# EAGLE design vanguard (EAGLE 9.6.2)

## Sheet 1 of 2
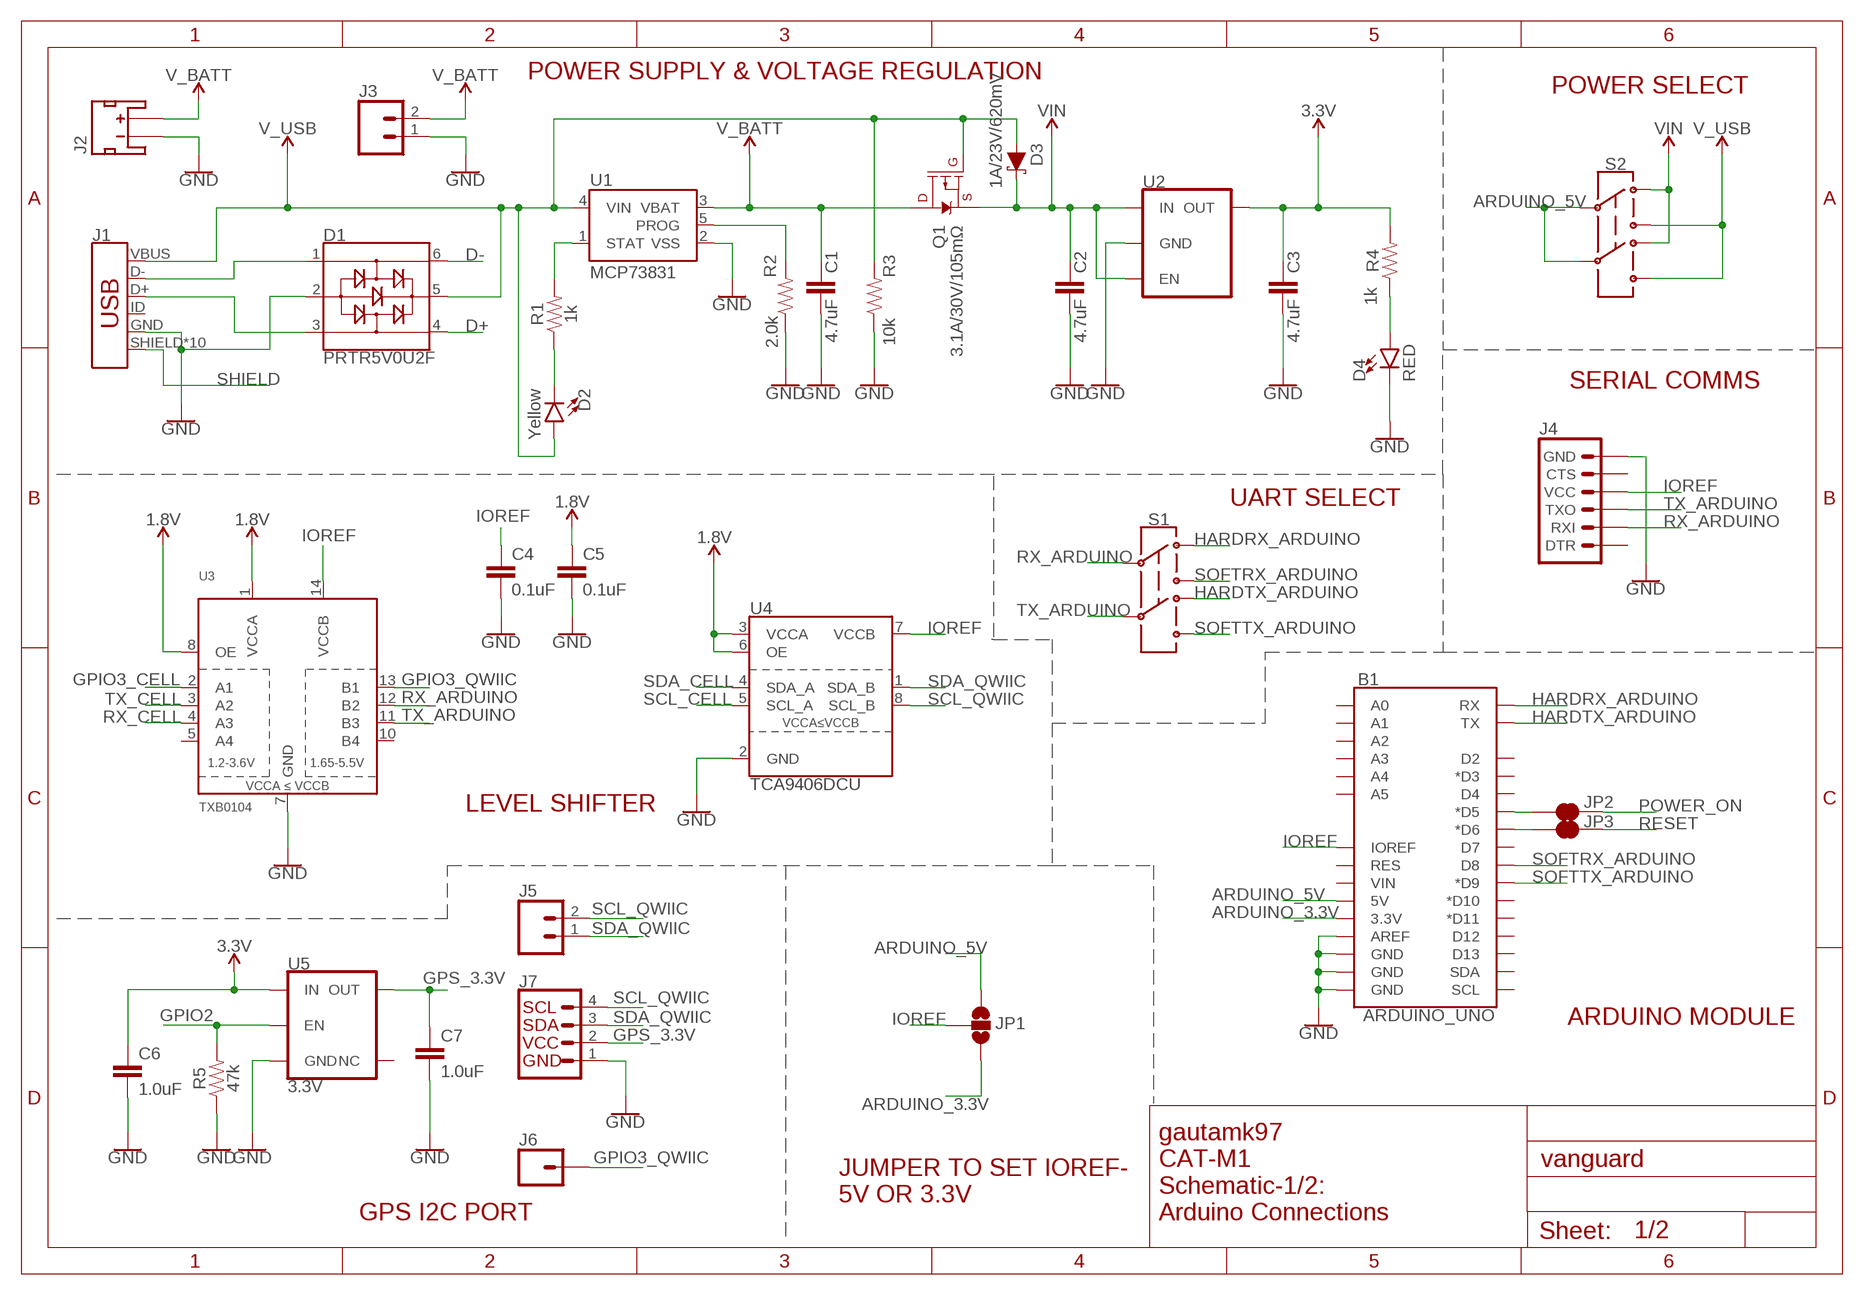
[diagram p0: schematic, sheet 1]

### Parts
B1  ARDUINO_UNO  ARDUINO_UNO_R3_SHIELDNOLABELS  [UNO_R3_SHIELD_NOLABELS]
C1  4.7uF  4.7UF-0603-6.3V-(10%)  [0603]
C2  4.7uF  4.7UF-0603-6.3V-(10%)  [0603]
C3  4.7uF  4.7UF-0603-6.3V-(10%)  [0603]
C4  0.1uF  0.1UF-0603-25V-(+80/-20%)  [0603]
C5  0.1uF  0.1UF-0603-25V-(+80/-20%)  [0603]
C6  1.0uF  1.0UF-0603-16V-10%  [0603]
C7  1.0uF  1.0UF-0603-16V-10%  [0603]
D1  PRTR5V0U2F  [SOT886]
D2  Yellow  LED-YELLOW0603  [LED-0603]
D3  1A/23V/620mV  DIODE-SCHOTTKY-BAT20J  [SOD-323]
D4  RED  LED-RED0603  [LED-0603]
J1  USB_MICRO-B_HALF_PTH_MILL  [USB-MICROB-PTH-MILL]
J2  JST_2MM_MALE  [JST-2-SMD]
J3  CONN_021X02_NO_SILK  [1X02_NO_SILK]
J4  6_PIN_SERIAL_TARGET_NO_SILK  [1X06_NO_SILK]
J5  CONN_021X02_NO_SILK  [1X02_NO_SILK]
J6  CONN_01PTH_NO_SILK_YES_STOP  [1X01_NO_SILK]
J7  QWIIC_CONNECTORJS-1MM  [JST04_1MM_RA]
JP1  JUMPER-SMT_3_NO_SILK  [SMT-JUMPER_3_NO_SILK]
JP2  JUMPER-SMT_2_NC_TRACE_SILK  [SMT-JUMPER_2_NC_TRACE_SILK]
JP3  JUMPER-SMT_2_NC_TRACE_SILK  [SMT-JUMPER_2_NC_TRACE_SILK]
Q1  3.1A/30V/105mΩ  MOSFET_PCH-DMG2307L  [SOT23-3]
R1  1k  1KOHM-0603-1/10W-1%  [0603]
R2  2.0k  2.0KOHM-0603-1/10W-5%  [0603]
R3  10k  10KOHM-0603-1/10W-1%  [0603]
R4  1k  1KOHM-0603-1/10W-1%  [0603]
R5  47k  47KOHM-0603-1/10W-1%  [0603]
S1  SWITCH-DPDT-SMD-AYZ0202  [SWITCH_DPDT_SMD_AYZ0202]
S2  SWITCH-DPDT-SMD-AYZ0202  [SWITCH_DPDT_SMD_AYZ0202]
U1  MCP73831  [SOT23-5]
U2  AP7361C-33FGEUDFN-8  [UDFN-8]
U3  TXB0104  TXB0104PWR  [TSSOP14]
U4  TCA9406DCU  [VSSOP-8]
U5  3.3V  V_REG_AP2112K-3.3V  [SOT23-5]

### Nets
1.8V: C5.1 U3.1(VCCA) U3.8(OE) U4.3(VCCA) U4.6(OE) ; also sheet 2
3.3V: C3.1 C6.1 R4.2 U2.1(OUT) U5.1(IN) ; also sheet 2
ARDUINO_3.3V: B1.3.3V JP1.3
ARDUINO_5V: B1.5V JP1.1 S2.2 S2.5
D+: D1.4 ; also sheet 2
D-: D1.6 ; also sheet 2
GND: B1.AREF B1.GND@0(GND) B1.GND@1(GND) B1.GND@2(GND) C1.2 C2.2 C3.2 C4.2 C5.2 C6.2 C7.2 D1.2 D4.C J1.GND J2.1(-) J3.1 J4.6(GND) J7.1 R2.1 R3.1 R5.1 U1.2(VSS) U2.4(GND) U2.EP(GND) U3.7(GND) U4.2(GND) U5.2(GND) ; also sheet 2
GPIO2: R5.2 U5.3(EN) ; also sheet 2
GPIO3_CELL: U3.2(A1)
GPIO3_QWIIC: J6.1 U3.13(B1)
GPS_3.3V: C7.1 J7.2 U5.5(OUT)
HARDRX_ARDUINO: B1.RX S1.3
HARDTX_ARDUINO: B1.TX S1.6
IOREF: B1.IOREF C4.1 J4.4(VCC) JP1.2 U3.14(VCCB) U4.7(VCCB)
N$1: D1.1 J1.D-
N$3: D1.3 J1.D+
N$4: D4.A R4.1
N$6: R1.2 U1.1(STAT)
N$7: D2.C R1.1
N$9: B1.D5(*D5) JP2.1
N$10: R2.2 U1.5(PROG)
N$11: B1.D6(*D6) JP3.1
POWER_ON: JP2.2
RESET: JP3.2
RX_ARDUINO: J4.2(RXI) S1.2 U3.12(B2)
RX_CELL: U3.4(A3) ; also sheet 2
SCL_CELL: U4.5(SCL_A) ; also sheet 2
SCL_QWIIC: J5.2 J7.4 U4.8(SCL_B)
SDA_CELL: U4.4(SDA_A) ; also sheet 2
SDA_QWIIC: J5.1 J7.3 U4.1(SDA_B)
SHIELD: J1.SHIELD J1.SHIELD2(SHIELD) J1.SHIELD3(SHIELD) J1.SHIELD4(SHIELD) J1.SHIELD5(SHIELD) J1.SHIELD6(SHIELD) J1.SHIELD7(SHIELD) J1.SHIELD8(SHIELD) J1.SHIELD9(SHIELD) J1.SHIELD10(SHIELD)
SOFTRX_ARDUINO: B1.D8 S1.1
SOFTTX_ARDUINO: B1.D9(*D9) S1.4
TX_ARDUINO: J4.3(TXO) S1.5 U3.11(B3)
TX_CELL: U3.3(A2) ; also sheet 2
V_BATT: C1.1 J2.2(+) J3.2 Q1.3(D) U1.3(VBAT)
V_USB: D1.5 D2.A D3.A J1.VBUS Q1.1(G) R3.2 S2.1 S2.4 U1.4(VIN) ; also sheet 2
VIN: C2.1 D3.C Q1.2(S) S2.3 S2.6 U2.5(EN) U2.8(IN)
Unconnected: B1.A0 B1.A1 B1.A2 B1.A3 B1.A4 B1.A5 B1.D2 B1.D3(*D3) B1.D4 B1.D7 B1.D10(*D10) B1.D11(*D11) B1.D12 B1.D13 B1.RES B1.SCL B1.SDA B1.VIN J1.ID J2.NC1(PAD1) J2.NC2(PAD2) J4.1(DTR) J4.5(CTS) U3.5(A4) U3.10(B4) U5.4(NC)

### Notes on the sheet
- POWER SUPPLY & VOLTAGE REGULATION
- POWER SELECT
- SERIAL COMMS
- UART SELECT
- LEVEL SHIFTER
- ARDUINO MODULE
- JUMPER TO SET IOREF- 
  5V OR 3.3V
- GPS I2C PORT
- gautamk97
  CAT-M1
  Schematic-1/2: 
  Arduino Connections

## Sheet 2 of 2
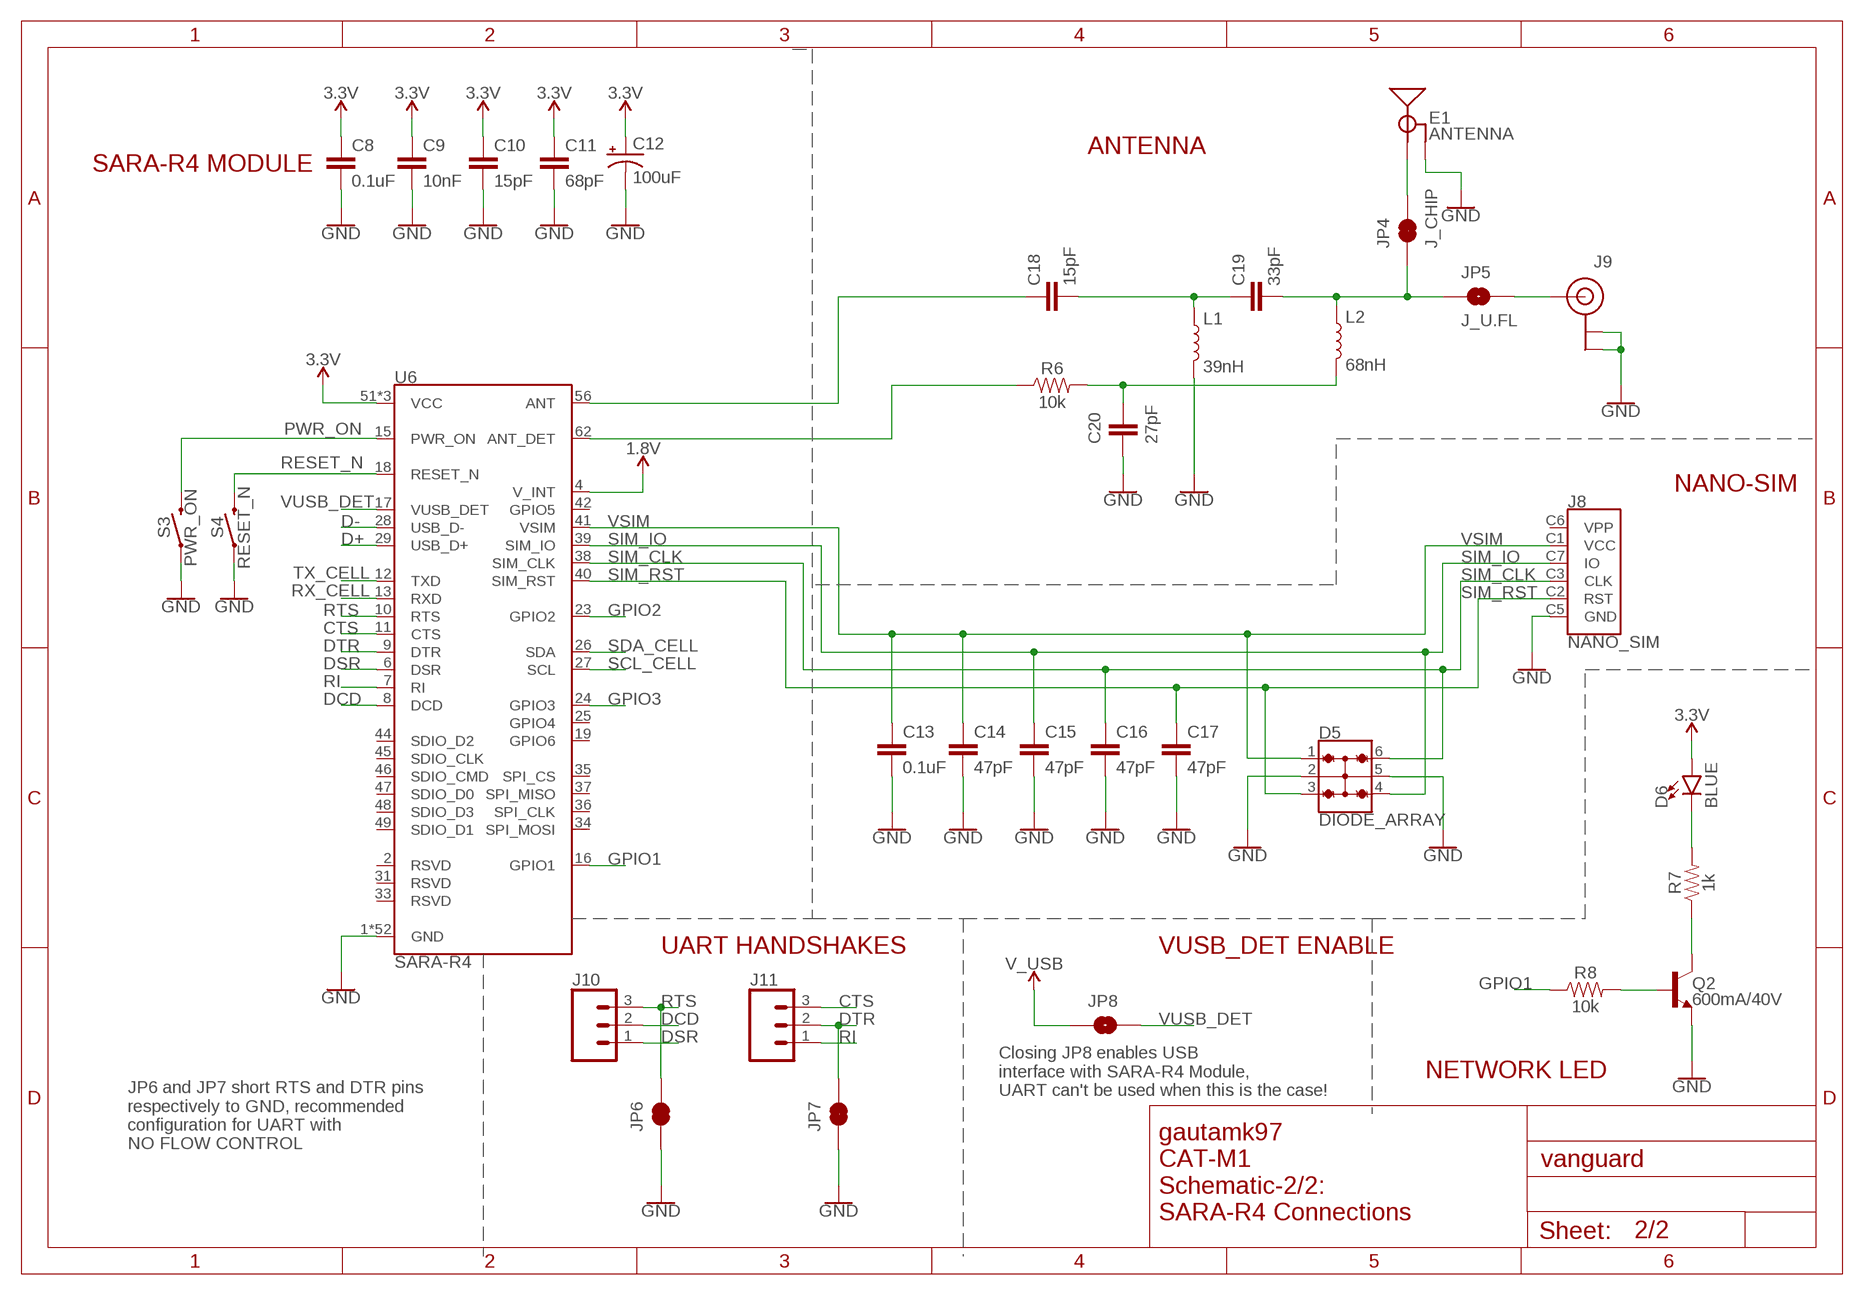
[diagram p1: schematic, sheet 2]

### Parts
C8  0.1uF  0.1UF-0603-25V-(+80/-20%)  [0603]
C9  10nF  10NF-0603-50V-10%  [0603]
C10  15pF  15PF-0603-50V-5%  [0603]
C11  68pF  68PF-0603-50V-5%  [0603]
C12  100uF  100UF-POLAR-1206-6.3V-20%  [1206-POLAR]
C13  0.1uF  0.1UF-0603-25V-(+80/-20%)  [0603]
C14  47pF  47PF-0603-50V-5%  [0603]
C15  47pF  47PF-0603-50V-5%  [0603]
C16  47pF  47PF-0603-50V-5%  [0603]
C17  47pF  47PF-0603-50V-5%  [0603]
C18  15pF  15PF-0603-50V-5%  [0603]
C19  33pF  33PF-0603-50V-5%  [0603]
C20  27pF  27PF-0603-50V-5%  [0603]
D5  DIODE_ARRAY  TVS_DIODE_ARRAY_4DT1042-04SO-7  [SOT23-6L]
D6  BLUE  LED-BLUE0603  [LED-0603]
E1  ANTENNA  ANTENNA-GROUNDEDMOLEX-146200  [MOLEX_146200]
J8  NANO_SIM  NANO_SIMWURTH  [NANO_SIM_WURTH_693043020611]
J9  U.FL  [U.FL]
J10  CONN_031X03_NO_SILK  [1X03_NO_SILK]
J11  CONN_031X03_NO_SILK  [1X03_NO_SILK]
JP4  J_CHIP  JUMPER-SMT_2_NC_TRACE_NO-SILK  [SMT-JUMPER_2_NC_TRACE_NO-SILK]
JP5  J_U.FL  JUMPER-SMT_2_NO_NO-SILK  [SMT-JUMPER_2_NO_NO-SILK]
JP6  JUMPER-SMT_2_NC_TRACE_SILK  [SMT-JUMPER_2_NC_TRACE_SILK]
JP7  JUMPER-SMT_2_NC_TRACE_SILK  [SMT-JUMPER_2_NC_TRACE_SILK]
JP8  JUMPER-SMT_2_NO_SILK  [SMT-JUMPER_2_NO_SILK]
L1  39nH  INDUCTOR-0603-39NH  [0603]
L2  68nH  INDUCTOR-0603-68NH  [0603]
Q2  600mA/40V  TRANS_NPN-MMBT2222AL  [SOT23-3]
R6  10k  10KOHM-0603-1/10W-1%  [0603]
R7  1k  1KOHM-0603-1/10W-1%  [0603]
R8  10k  10KOHM-0603-1/10W-1%  [0603]
S3  PWR_ON  MOMENTARY-SWITCH-SPST-SMD-5.2MM-TALL  [TACTILE_SWITCH_SMD_5.2MM]
S4  RESET_N  MOMENTARY-SWITCH-SPST-SMD-5.2MM-TALL  [TACTILE_SWITCH_SMD_5.2MM]
U6  SARA-R4  [SARA-LGA]

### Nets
1.8V: U6.4(V_INT) ; also sheet 1
3.3V: C8.1 C9.1 C10.1 C11.1 C12.1(+) D6.A U6.51(VCC) U6.52(VCC) U6.53(VCC) ; also sheet 1
CTS: J11.3 U6.11(CTS)
D+: U6.29(USB_D+) ; also sheet 1
D-: U6.28(USB_D-) ; also sheet 1
DCD: J10.2 U6.8(DCD)
DSR: J10.1 U6.6(DSR)
DTR: J11.2 JP7.2 U6.9(DTR)
GND: C8.2 C9.2 C10.2 C11.2 C12.2(-) C13.2 C14.2 C15.2 C16.2 C17.2 C20.2 D5.2 D5.5 E1.GND J8.C5(GND) J9.1(GND) J9.2(GND) JP6.1 JP7.1 L1.2 Q2.2(E) S3.1 S4.1 U6.1(GND) U6.3(GND) U6.5(GND) U6.14(GND) U6.20(GND) U6.21(GND) U6.22(GND) U6.30(GND) U6.32(GND) U6.43(GND) U6.50(GND) U6.54(GND) U6.55(GND) U6.57(GND) U6.58(GND) U6.59(GND) U6.60(GND) U6.61(GND) U6.63(GND) U6.64(GND) U6.65(GND) U6.66(GND) U6.67(GND) U6.68(GND) U6.69(GND) U6.70(GND) U6.71(GND) U6.72(GND) U6.73(GND) U6.74(GND) U6.75(GND) U6.76(GND) U6.77(GND) U6.78(GND) U6.79(GND) U6.80(GND) U6.81(GND) U6.82(GND) U6.83(GND) U6.84(GND) U6.85(GND) U6.86(GND) U6.87(GND) U6.88(GND) U6.89(GND) U6.90(GND) U6.91(GND) U6.92(GND) U6.93(GND) U6.94(GND) U6.95(GND) U6.96(GND) ; also sheet 1
GPIO1: R8.1 U6.16(GPIO1)
GPIO2: U6.23(GPIO2) ; also sheet 1
GPIO3: U6.24(GPIO3)
N$8: R6.1 U6.62(ANT_DET)
N$12: C18.1 U6.56(ANT)
N$13: C18.2 C19.1 L1.1
N$14: C20.1 L2.2 R6.2
N$15: C19.2 JP4.1 JP5.1 L2.1
N$16: E1.FEED(SIGNAL) JP4.2
N$17: D6.C R7.2
N$18: J9.FEED(SIGNAL) JP5.2
N$19: Q2.1(B) R8.2
N$20: Q2.3(C) R7.1
PWR_ON: S3.3 U6.15(PWR_ON)
RESET_N: S4.3 U6.18(RESET_N)
RI: J11.1 U6.7(RI)
RTS: J10.3 JP6.2 U6.10(RTS)
RX_CELL: U6.13(RXD) ; also sheet 1
SCL_CELL: U6.27(SCL) ; also sheet 1
SDA_CELL: U6.26(SDA) ; also sheet 1
SIM_CLK: C16.1 D5.6 J8.C3(CLK) U6.38(SIM_CLK)
SIM_IO: C15.1 D5.4 J8.C7(IO) U6.39(SIM_IO)
SIM_RST: C17.1 D5.3 J8.C2(RST) U6.40(SIM_RST)
TX_CELL: U6.12(TXD) ; also sheet 1
V_USB: JP8.1 ; also sheet 1
VSIM: C13.1 C14.1 D5.1 J8.C1(VCC) U6.41(VSIM)
VUSB_DET: JP8.2 U6.17(VUSB_DET)
Unconnected: J8.C6(VPP) U6.2(RSVD) U6.19(GPIO6) U6.25(GPIO4) U6.31(RSVD) U6.33(RSVD) U6.34(SPI_MOSI) U6.35(SPI_CS) U6.36(SPI_CLK) U6.37(SPI_MISO) U6.42(GPIO5) U6.44(SDIO_D2) U6.45(SDIO_CLK) U6.46(SDIO_CMD) U6.47(SDIO_D0) U6.48(SDIO_D3) U6.49(SDIO_D1)

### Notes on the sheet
- ANTENNA
- SARA-R4 MODULE
- NANO-SIM
- UART HANDSHAKES | VUSB_DET ENABLE
- NETWORK LED
- Closing JP8 enables USB 
  interface with SARA-R4 Module, 
  UART can't be used when this is the case!
- JP6 and JP7 short RTS and DTR pins 
  respectively to GND, recommended 
  configuration for UART with 
  NO FLOW CONTROL
- gautamk97
  CAT-M1
  Schematic-2/2:
  SARA-R4 Connections

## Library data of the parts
B1 = SparkFun-Boards:ARDUINO_UNO_R3_SHIELD: Arduino R3 Shield Footprint Shield form compatible with the Arduino Uno R3. SparkFun Products: MG2639 Cellular Shield MIDI Shield R3 Stackable Headers Kit
C1-C3 = SparkFun-Capacitors:4.7UF: 4.7µF ceramic capacitors; PROD_ID: CAP-08280
C4 C5 C8 C13 = SparkFun-Capacitors:0.1UF: 0.1µF ceramic capacitors; PROD_ID: CAP-00810
C6 C7 = SparkFun-Capacitors:1.0UF: 1µF ceramic capacitors; PROD_ID: CAP-00868
C9 = SparkFun-Capacitors:10NF: 0.01uF/10nF/10,000pF ceramic capacitors; PROD_ID: CAP-00867
C10 C18 = SparkFun-Capacitors:15PF: 15pF ceramic capacitors; PROD_ID: CAP-07881
C11 = SparkFun-Capacitors:68PF: 68pF ceramic capacitors; PROD_ID: CAP-14092
C12 = ublox:100UF-POLAR: 100µF polarized capacitors; PROD_ID: CAP-14093
C14-C17 = SparkFun-Capacitors:47PF: 47pF ceramic capacitors; PROD_ID: CAP-08913
C19 = SparkFun-Capacitors:33PF: 33pF ceramic capacitors; PROD_ID: CAP-10142
C20 = SparkFun-Capacitors:27PF: 27pF ceramic capacitors; PROD_ID: CAP-09989
D1 = SparkFun-IC-Power:PRTR5V0U2: A small ESD protection device. Most commonly used on USB D+/D- signals to protect large, expensive, or especially sensitive USB enabled devices.; PROD_ID: DIO-14084
D2 = SparkFun-LED:LED-YELLOW: Yellow SMD LED; PROD_ID: DIO-09003
D3 = SparkFun-DiscreteSemi:DIODE-SCHOTTKY: Schottky diode; PROD_ID: DIO-11623
D4 = SparkFun-LED:LED-RED: Red SMD LED; PROD_ID: DIO-00819
D5 = ublox:TVS_DIODE_ARRAY_4; PROD_ID: DIO-14095
D6 = SparkFun-LED:LED-BLUE: Blue SMD LED; PROD_ID: DIO-08575
E1 = ublox:ANTENNA-GROUNDED: Antenna w/ Ground Connection; PROD_ID: ANT-14096
J1 = SparkFun-Connectors:USB_MICRO-B: USB Type Micro-B Connector Male/female and PTH/SMT variants SparkFun Products: SparkFun microB USB Breakout SparkFun USB microB Plug Breakout SparkFun ESP8266 Thing; PROD_ID: CONN-13711
J2 = SparkFun-Connectors:JST_2MM_MALE: JST 2MM MALE RA CONNECTOR Two pin, compact surface mount connector. Commonly used as a battery input connection point. We really like the solid locking feeling and high current rating on these small connectors. We use these all the time as battery connectors. Mates to single-cell LiPo batteries.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; PROD_ID: CONN-11443; SF_ID: PRT-08612
J3 J5 = SparkFun-Connectors:CONN_02: Multi connection point. Often used as Generic Header-pin footprint for 0.1 inch spaced/style header connections
J4 = SparkFun-Connectors:6_PIN_SERIAL_TARGET: 6-pin header connection for use with the "FTDI BASIC" pinout - TARGET SIDE. Also known as "Arduino Serial Program Header". It is used to mate with our FTDI Basic serial programmers using the Arduino IDE. Note, this device has "TARGET" in the name. It is intended to be used on a design that contains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
J6 = SparkFun-Connectors:CONN_01: Single connection point. Often used as Generic Header-pin footprint for 0.1 inch spaced/style header connections
J7 = SparkFun-Connectors:QWIIC_CONNECTOR: SparkFun I2C Standard Qwiic Connector An SMD 1mm pitch JST connector makes it easy and quick (get it? Qwiic?) to connect I2C devices to each other. The Qwiic system enables fast and solderless connection between popular platforms and various sensors and actuators. We carry 200mm, 100mm, 50mm, and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; PROD_ID: CONN-13694; VALUE: QWIIC_RIGHT_ANGLE
J8 = ublox:NANO_SIM; PROD_ID: CONN-14097
J9 = SparkFun-Connectors:U.FL: SMD Antenna Connector - U.FL 2mm height, 3.0mm x 3.0mm receptacle size. SparkFun Products: SparkFun WiFi Shield - ESP8266 SparkFun ESP8266 Thing SparkFun MiniGen - Pro Mini Signal Generator Shield; PROD_ID: CONN-09193; SF_ID: WRL-09144
J10 J11 = SparkFun-Connectors:CONN_03: Multi connection point. Often used as Generic Header-pin footprint for 0.1 inch spaced/style header connections On any of the 0.1 inch spaced packages, you can populate with these: Break Away Headers - Straight (PRT-00116) Break Away Male Headers - Right Angle (PRT-00553) Female Headers (PRT-00115)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
JP1 = SparkFun-Jumpers:JUMPER-SMT_3_NO: Normally open jumper This jumper has three pads in close proximity to each other. Apply solder to close the connection(s).
JP2-JP4 JP6 JP7 = SparkFun-Jumpers:JUMPER-SMT_2_NC_TRACE: Normally closed trace jumper
JP5 JP8 = SparkFun-Jumpers:JUMPER-SMT_2_NO: Normally open jumper
L1 = ublox:INDUCTOR: Inductors; PROD_ID: NDUC-14091
L2 = ublox:INDUCTOR: Inductors
Q1 = SparkFun-DiscreteSemi:MOSFET_PCH: P-channel MOSFETs Voltage controlled devices that allow control of high current outputs. SparkFun Products: SparkFun ESP32 Thing SparkFun ESP8266 Thing SparkFun Pi Servo HAT V2 DMG2305UX-7 (20V/4.2A/SOT23-3); PROD_ID: TRANS-11308
Q2 = SparkFun-DiscreteSemi:TRANS_NPN: NPN transistor Current controlled devices typically used to amplify current or used as a switch. BC547 - COM-08928 (TO-92 45V 100mA) (1.Collector 2.Base 3.Emitter) 2N3904 - COM-00521 (TO-92 40V 200mA) (1.Emitter 2.Base 3.Collector) P2N2222A - COM-12852 (TO-92 40V 600mA) (1.Collector 2.Base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; PROD_ID: TRANS-08049
R1 R4 R7 = SparkFun-Resistors:1KOHM: 1kΩ resistor; PROD_ID: RES-07856
R2 = SparkFun-Resistors:2.0KOHM: 2kΩ resistor; PROD_ID: RES-08296
R3 R6 R8 = SparkFun-Resistors:10KOHM: 10kΩ resistor; PROD_ID: RES-00824
R5 = SparkFun-Resistors:47KOHM: 47kΩ resistor; PROD_ID: RES-07871
S1 S2 = SparkFun-Switches:SWITCH-DPDT: Double-Pole, Double-Throw (DPDT) Switch Double-pole, double-throw switches. Variant Overview PTH-GPI-152-3013 Used on SparkFun Geiger Counter SMD-AY0202 Surface Mount DPDT Switch (COM-00597) Used on e.g. LilyPad Arduino USB - ATmega32U4 Board; PROD_ID: SWCH-08179; SF_SKU: COM-00597
S3 S4 = SparkFun-Switches:MOMENTARY-SWITCH-SPST: Momentary Switch (Pushbutton) - SPST; PROD_ID: SWCH-14139
U1 = SparkFun-IC-Power:MCP73831: MCP73831T Li-Ion, Li-Pol Controller Miniature single cell, fully integrated Li-Ion, Li-polymer charge management controller Datasheet SparkFun Products: SparkFun ESP32 Thing SparkFun 9DoF Razor IMU M0; PROD_ID: IC-09995
U2 = SparkFun-IC-Power:AP7361C-33FGE: AP7361C 3.3V LDO Regulator; PROD_ID: VREG-14094
U3 = SparkFun-IC-Comms:TXB0104PWR: 4-Bit Bi-Directional Level Shifter 1.2V-3.6V (VCCA) to 1.65V-5.5V (VCCB) bi-directional level shifter with auto direction sensing. Max data rate - VCCA 1.8V: 20Mbps (50ns), VCCA 3.3V: 100Mbps (10ns) Digikey: 296-21929-1-ND (TSSOP) Datasheet SparkFun Products SparkFun Cellular Shield - MG2639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; PROD_ID: IC-13929
U4 = ublox:TCA9406; PROD_ID: IC-14098
U5 = SparkFun-IC-Power:V_REG_AP2112: AP2112 - 600mA CMOS LDO Regulator w/ Enable The AP2112 is CMOS process low dropout linear regulator with enable function, the regulator delivers a guaranteed 600mA (min.) continuous load current. Features Output Voltage Accuracy: ±1.5% Output Current: 600mA (Min.) Foldback Short Current Protection: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; PROD_ID: VREG-12457
U6 = ublox:SARA-R4; PROD_ID: IC-14085

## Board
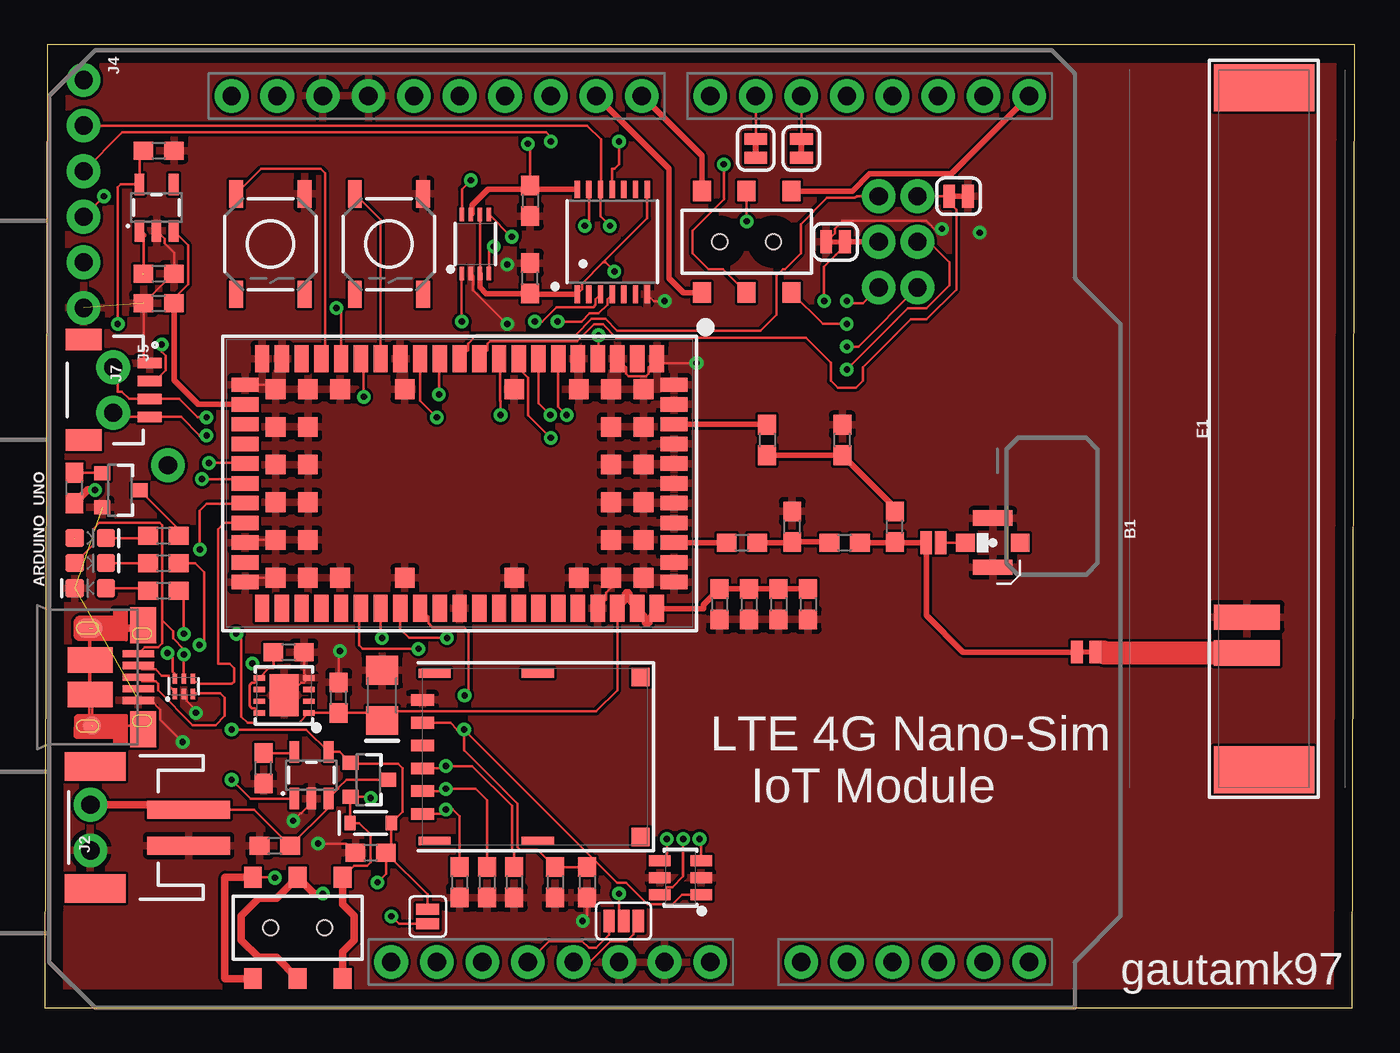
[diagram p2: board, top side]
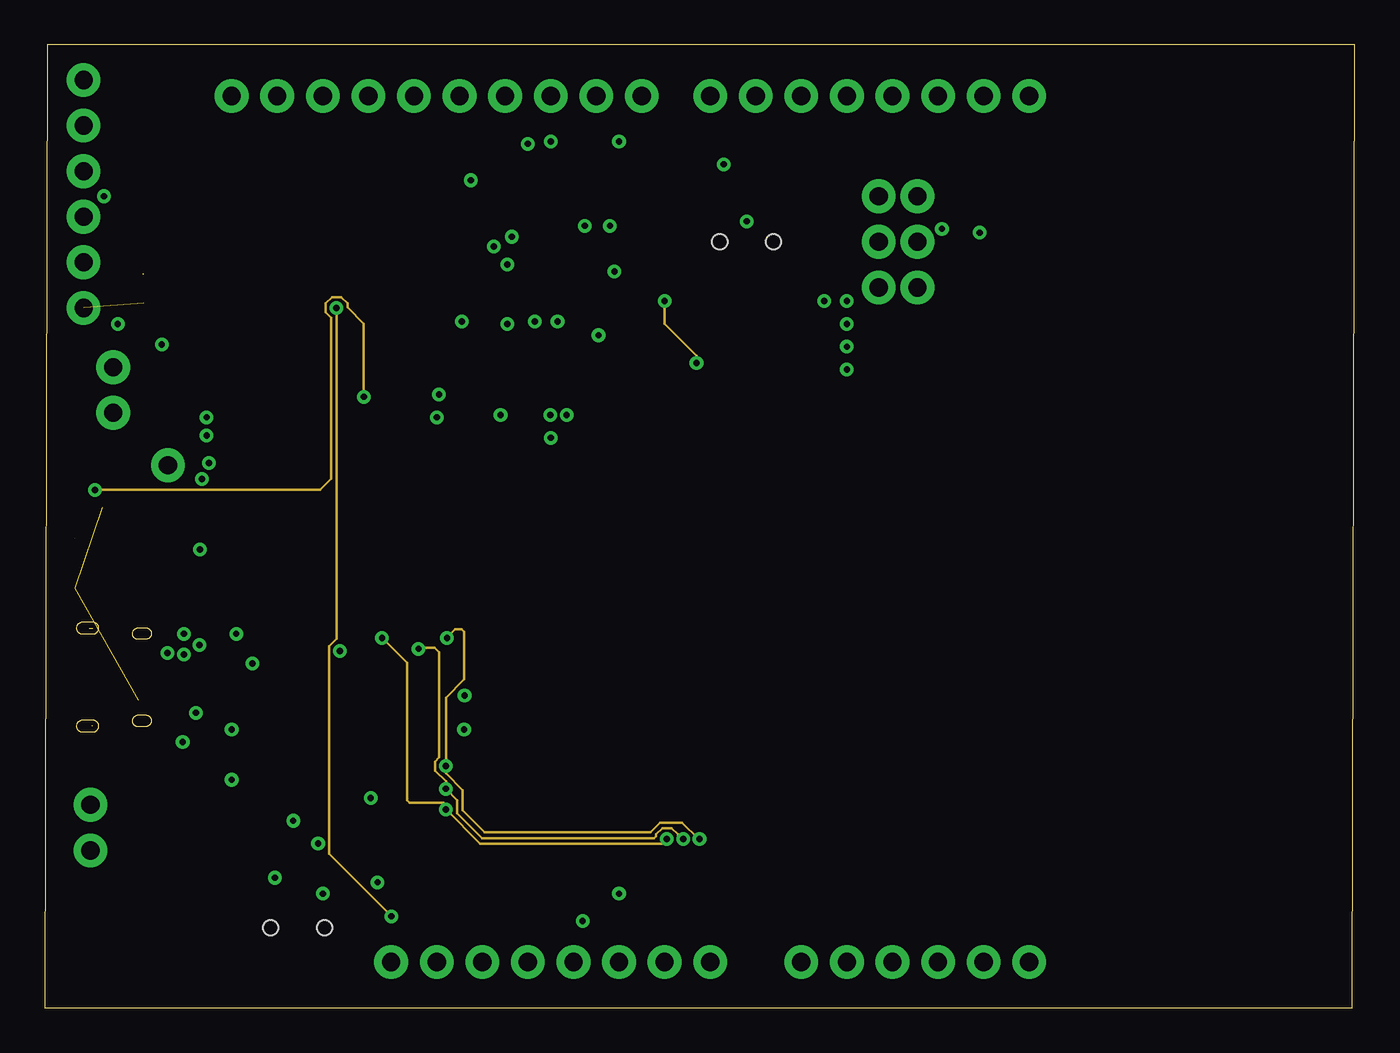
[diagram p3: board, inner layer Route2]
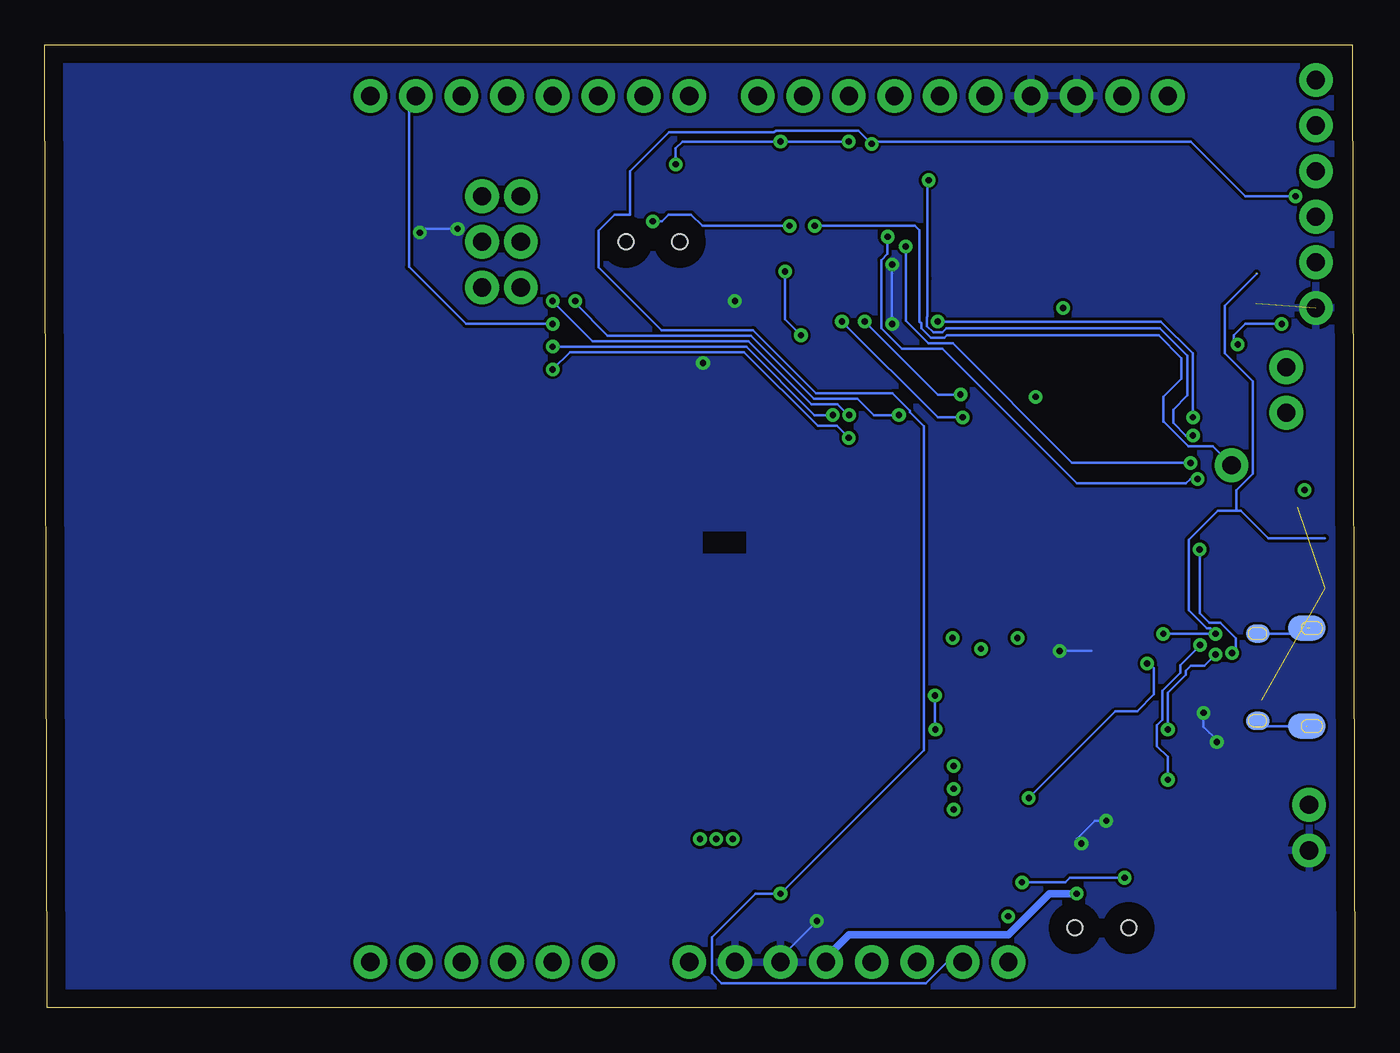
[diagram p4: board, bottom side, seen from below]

Size 73.01 x 53.65 mm. Coordinates in mm from the lower left corner, seen from the top.
Outline: 0,0 72.88,0 73.01,53.65 0.13,53.65 0,0
Copper layers (1*16): Top 0.035mm / dielectric 1.5mm / Bottom 0.035mm
Design rules "default": minimum track width 6mil, minimum drill 0.35mm, track to track 6mil, track to pad 6mil, pad to pad 6mil, via to via 6mil, smd to smd 6mil, copper to edge 40mil, drill to drill 6mil, minimum pad ring 10mil, minimum via ring 8mil, stop-mask expansion 4mil, vias tented up to drill 0mil, thermal gap 10mil

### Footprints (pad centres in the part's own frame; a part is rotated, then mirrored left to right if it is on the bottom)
UNO_R3_SHIELD_NOLABELS = drill 1.016 pad 1.88: 3.3V 24.13,-3.81; 5V 24.13,-1.27; A0 24.13,11.43; A1 24.13,13.97; A2 24.13,16.51; A3 24.13,19.05; A4 24.13,21.59; A5 24.13,24.13; AREF -24.13,-15.24; D2 -24.13,19.05; D3 -24.13,16.51; D4 -24.13,13.97; D5 -24.13,11.43; D6 -24.13,8.89; D7 -24.13,6.35; D8 -24.13,2.54; D9 -24.13,0; D10 -24.13,-2.54; D11 -24.13,-5.08; D12 -24.13,-7.62; D13 -24.13,-10.16; GND@0 24.13,1.27; GND@1 24.13,3.81; GND@2 -24.13,-12.7; IOREF 24.13,-8.89; NC 24.13,-11.43; RES 24.13,-6.35; RX -24.13,24.13; SCL -24.13,-20.32; SDA -24.13,-17.78; TX -24.13,21.59; VIN 24.13,6.35
0603 = smd 1.1 x 1: 1 -0.85,0; 2 0.85,0
1206-POLAR = smd 1.6 x 1.8: 1 -1.4,0; 2 1.4,0
SOT886 = smd 0.61 x 0.25: 1 -0.405,0.5 | smd 0.56 x 0.25: 2 -0.43,0; 3 -0.43,-0.5; 4 0.43,-0.5; 5 0.43,0; 6 0.43,0.5
LED-0603 = smd 1 x 1: A -0.877,0; C 0.877,0
SOD-323 = smd 0.63 x 0.83: A 1.15,0; C -1.15,0
SOT23-6L = smd 0.6 x 1.2: 1 -0.95,-1.15; 2 0,-1.15; 3 0.95,-1.15; 4 0.95,1.15; 5 0,1.15; 6 -0.95,1.15
MOLEX_146200 = smd 1.4 x 3.7: FEED 12.5,-0.95; GND 10.5,-0.95 | smd 2.6 x 5.6: MNT1 -19,0; MNT2 19,0
USB-MICROB-PTH-MILL = smd 0.4 x 1.75: D+ 0,0; D- -0.65,0; GND 1.3,0; ID 0.65,0; VBUS -1.3,0 | smd 2 x 1.46: SHIELD -2.9,0.275; SHIELD2 2.9,0.275 | smd 1.425 x 2.5: SHIELD3 -0.963,-2.675; SHIELD4 0.963,-2.675 | smd 1.4 x 2.1 bottom: SHIELD5 -2.731,-2.531; SHIELD7 2.729,-2.531 | smd 1 x 1: SHIELD6 2.7,-2.575 | smd 1.1 x 1.5: SHIELD8 -2.731,-2.731 | smd 1 x 1.3 bottom: SHIELD9 -2.43,0.195; SHIELD10 2.43,0.195
JST-2-SMD = smd 1 x 4.6: 1 -1,-3.7; 2 1,-3.7 | smd 1.6 x 3.4: NC1 -3.4,1.5; NC2 3.4,1.5
1X02_NO_SILK = drill 1.016 pad 1.88: 1 0,0; 2 2.54,0
1X06_NO_SILK = drill 1.016 pad 1.88: 1 0,0; 2 2.54,0; 3 5.08,0; 4 7.62,0; 5 10.16,0; 6 12.7,0
1X01_NO_SILK = drill 1.016 pad 1.88: 1 0,0
JST04_1MM_RA = smd 0.6 x 1.35: 1 -1.5,0; 2 -0.5,0; 3 0.5,0; 4 1.5,0 | smd 1.2 x 2: NC1 2.8,-3.675; NC2 -2.8,-3.675
NANO_SIM_WURTH_693043020611 = smd 0.65 x 1.3: C1 1.905,6.25; C2 -0.635,6.25; C3 -1.905,6.25; C5 3.175,6.25; C6 0.635,6.25; C7 -3.175,6.25 | smd 0.48 x 1.8: MNT1 -4.69,5.58; MNT2 4.66,5.58; MNT3 -4.69,-0.17; MNT4 4.66,-0.17 | smd 1.03 x 1: MNT5 -4.465,-5.89; MNT6 4.465,-5.89
U.FL = smd 2.2 x 0.85: 1 0,1.375; 2 0,-1.375 | smd 1.05 x 1: FEED 1.525,0; NC -1.525,0
1X03_NO_SILK = drill 1.016 pad 1.88: 1 0,0; 2 2.54,0; 3 5.08,0
SMT-JUMPER_3_NO_SILK = smd 0.635 x 1.27: 1 -0.813,0; 2 0,0; 3 0.813,0
SMT-JUMPER_2_NC_TRACE_SILK = smd 0.66 x 1.27: 1 -0.521,0; 2 0.521,0
SMT-JUMPER_2_NC_TRACE_NO-SILK = smd 0.66 x 1.27: 1 -0.521,0; 2 0.521,0
SMT-JUMPER_2_NO_NO-SILK = smd 0.635 x 1.27: 1 -0.406,0; 2 0.406,0
SMT-JUMPER_2_NO_SILK = smd 0.635 x 1.27: 1 -0.406,0; 2 0.406,0
SOT23-3 = smd 0.8 x 0.9: 1 -0.95,-1; 2 0.95,-1; 3 0,1.1
SWITCH_DPDT_SMD_AYZ0202 = smd 1 x 1.15: 1 -2.5,2.825; 2 0,2.825; 3 2.5,2.825; 4 -2.5,-2.825; 5 0,-2.825; 6 2.5,-2.825 | hole 0.85: 1.5,0; -1.5,0
TACTILE_SWITCH_SMD_5.2MM = smd 1.524 x 0.762: 1 -2.794,1.905; 2 2.794,1.905; 3 -2.794,-1.905; 4 2.794,-1.905
SOT23-5 = smd 0.55 x 1.2: 1 -0.95,-1.3; 2 0,-1.3; 3 0.95,-1.3; 4 0.95,1.3; 5 -0.95,1.3
UDFN-8 = smd 0.3 x 0.65: 1 -0.975,-1.375; 2 -0.325,-1.375; 3 0.325,-1.375; 4 0.975,-1.375; 5 0.975,1.375; 6 0.325,1.375; 7 -0.325,1.375; 8 -0.975,1.375 | smd 2.35 x 1.6: EP 0,0
TSSOP14 = smd 0.305 x 0.991: 1 -1.95,-2.918; 2 -1.3,-2.918; 3 -0.65,-2.918; 4 0,-2.918; 5 0.65,-2.918; 6 1.3,-2.918; 7 1.95,-2.918; 8 1.95,2.918; 9 1.3,2.918; 10 0.65,2.918; 11 0,2.918; 12 -0.65,2.918; 13 -1.3,2.918; 14 -1.95,2.918
VSSOP-8 = smd 0.75 x 0.25: 1 -1.65,0.75; 2 -1.65,0.25; 3 -1.65,-0.25; 4 -1.65,-0.75; 5 1.65,-0.75; 6 1.65,-0.25; 7 1.65,0.25; 8 1.65,0.75
SARA-LGA = smd 0.8 x 1.5: 1 -11,-6.95; 2 -9.9,-6.95; 3 -8.8,-6.95; 4 -7.7,-6.95; 5 -6.6,-6.95; 6 -5.5,-6.95; 7 -4.4,-6.95; 8 -3.3,-6.95; 9 -2.2,-6.95; 10 -1.1,-6.95; 11 0,-6.95; 12 1.1,-6.95; 13 2.2,-6.95; 14 3.3,-6.95; 15 4.4,-6.95; 16 5.5,-6.95; 17 6.6,-6.95; 18 7.7,-6.95; 19 8.8,-6.95; 20 9.9,-6.95; 21 11,-6.95; 33 11,6.95; 34 9.9,6.95; 35 8.8,6.95; 36 7.7,6.95; 37 6.6,6.95; 38 5.5,6.95; 39 4.4,6.95; 40 3.3,6.95; 41 2.2,6.95; 42 1.1,6.95; 43 0,6.95; 44 -1.1,6.95; 45 -2.2,6.95; 46 -3.3,6.95; 47 -4.4,6.95; 48 -5.5,6.95; 49 -6.6,6.95; 50 -7.7,6.95; 51 -8.8,6.95; 52 -9.9,6.95; 53 -11,6.95 | smd 1.5 x 0.8: 22 11.95,-5.5; 23 11.95,-4.4; 24 11.95,-3.3; 25 11.95,-2.2; 26 11.95,-1.1; 27 11.95,0; 28 11.95,1.1; 29 11.95,2.2; 30 11.95,3.3; 31 11.95,4.4; 32 11.95,5.5; 54 -11.95,5.5; 55 -11.95,4.4; 56 -11.95,3.3; 57 -11.95,2.2; 58 -11.95,1.1; 59 -11.95,0; 60 -11.95,-1.1; 61 -11.95,-2.2; 62 -11.95,-3.3; 63 -11.95,-4.4; 64 -11.95,-5.5 | smd 1.1 x 1.1: 65 -10.25,-5.25; 66 -10.25,-3.15; 67 -10.25,-1.05; 68 -10.25,1.05; 69 -10.25,3.15; 70 -10.25,5.25; 71 -8.45,-5.25; 72 -8.45,-3.15; 73 -8.45,-1.05; 74 -8.45,1.05; 75 -8.45,3.15; 76 -8.45,5.25; 77 -6.65,-5.25; 78 -6.65,5.25; 79 -3.05,-5.25; 80 -3.05,5.25; 81 3.05,-5.25; 82 3.05,5.25; 83 6.65,-5.25; 84 6.65,5.25; 85 8.45,-5.25; 86 8.45,-3.15; 87 8.45,-1.05; 88 8.45,1.05; 89 8.45,3.15; 90 8.45,5.25; 91 10.25,-5.25; 92 10.25,-3.15; 93 10.25,-1.05; 94 10.25,1.05; 95 10.25,3.15; 96 10.25,5.25

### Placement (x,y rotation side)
B1  30.73,26.67 270 top
C1  12.83,9.02 180 top
C2  13.59,19.81 0 top
C3  16.38,17.27 90 top
C4  27.05,44.96 270 top
C5  27.05,40.64 90 top
C6  6.35,40.89 0 top
C7  6.35,47.75 0 top
C8  37.59,22.48 270 top
C9  39.24,22.48 270 top
C10  40.89,22.48 270 top
C11  42.54,22.48 270 top
C12  18.8,17.4 90 top
C13  28.45,6.99 270 top
C14  30.23,6.99 270 top
C15  23.11,6.99 270 top
C16  24.64,6.99 270 top
C17  26.16,6.99 270 top
C18  38.86,25.91 0 top
C19  44.58,25.91 0 top
C20  44.45,31.62 90 top
D1  7.75,17.91 90 top
D2  2.54,24.77 0 top
D3  18.16,10.29 0 top
D4  2.54,23.37 180 top
D5  35.43,7.24 90 top
D6  2.54,26.16 0 top
E1  67.95,32.26 270 top
J1  5.21,18.41 270 top
J2  4.32,10.03 90 top
J3  2.54,8.76 90 top
J4  2.16,51.69 270 top
J5  3.81,35.69 270 top
J6  6.86,30.23 0 top
J7  5.84,34.42 270 top
J8  27.3,13.97 90 top
J9  52.83,25.91 180 top
J10  48.64,40.13 90 top
J11  46.48,40.13 90 top
JP1  32.26,4.83 180 top
JP2  42.16,47.88 270 top
JP3  39.62,47.88 270 top
JP4  58.04,19.81 0 top
JP5  49.53,25.91 0 top
JP6  50.93,45.21 180 top
JP7  44.07,42.67 0 top
JP8  21.34,5.08 270 top
L1  41.66,26.8 90 top
L2  47.37,26.8 90 top
Q1  18.03,12.7 270 top
Q2  4.19,28.83 270 top
R1  6.6,24.77 0 top
R2  12.19,13.34 90 top
R3  18.16,8.64 0 top
R4  6.6,23.24 0 top
R5  6.35,39.24 0 top
R6  40.26,31.62 270 top
R7  6.6,26.29 180 top
R8  1.65,28.96 90 top
S1  39.12,42.67 0 top
S2  14.1,4.45 0 top
S3  19.18,42.55 270 top
S4  12.57,42.55 270 top
U1  14.86,12.95 0 top
U2  13.33,17.4 90 top
U3  31.62,42.67 0 top
U4  24,42.55 90 top
U5  6.22,44.58 0 top
U6  23.11,29.21 180 top

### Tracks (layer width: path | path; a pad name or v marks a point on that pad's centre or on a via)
1.8V  (via drill 0.35)
  Top 0.152: U4.3 U4.6 | U3.1 29.94,40.02 29.94,40.34 31.12,41.52 | U3.8 33.57,43.98 31.12,41.52 | 31.12,41.52 31.25,41.52 v31.75,41.02 | v30.86,37.47 30.86,36.21 U6.4
  Top 0.305: U3.1 27.09,39.75 C5.1 24.6,39.79 24.25,40.14 U4.3
  Bottom 0.152: v31.75,41.02 31.75,38.35 v30.86,37.47
3.3V  (via drill 0.35)  (2 unrouted)
  Top 0.152: U6.51 31.91,17.69 30.73,16.51 19.31,16.51 C12.1 18.37,16.42 C3.1 U2.1 14.16,15.88 11.3,15.88 10.96,16.22 10.96,20.54 v10.67,20.83 | v7.75,20.83 7.75,22.95 R4.2 | 5.5,43.05 C6.1
  Top 0.305: C11.1 C10.1 C9.1 C8.1 36.7,22.44 36.7,22.23 34.15,22.23 | 34.15,22.23 U6.53 | U6.51 32.31,22.66 32.31,23.07 32.4,23.16 32.53,23.16 32.62,23.07 32.62,22.66 U6.52 33.41,21.86 33.41,21.45 33.5,21.36 33.63,21.36 33.72,21.45 33.72,21.79 34.15,22.23 | U5.1 5.5,43.05
  Bottom 0.152: v10.67,20.83 v7.75,20.83 8.05,21.13 8.23,21.13 9.24,22.15 9.24,26.06 7.62,27.69 6.6,27.69 | 6.6,27.69 6.35,27.69 4.83,26.16 1.65,26.16 | 6.6,27.69 6.6,28.83 5.69,29.74 5.69,34.9 7.24,36.45 7.24,39.12 5.46,40.89
ARDUINO_3.3V
  Top 0.152: B1.3.3V 28.09,3.71 29.95,3.71 30.33,3.33 30.71,3.33 31.45,4.07 JP1.3
ARDUINO_5V  (via drill 0.35)
  Top 0.152: JP1.1 32.8,4.56 32.8,4.1 32.42,3.71 31.52,3.71 30.35,2.54 B1.5V
  Top 0.406: S2.5 12.92,2.8 11.92,2.8 10.95,3.76 10.95,5.13 11.92,6.09 12.92,6.09 S2.2 15.02,6.35 v15.49,6.35
  Bottom 0.406: v15.49,6.35 17.02,6.35 19.3,4.06 28.19,4.06 29.46,2.79 B1.5V
CTS
  Top 0.152: U6.11 23.59,36.63 23.59,37.01 24.05,37.47 29.57,37.47 30.48,38.38 31.24,38.38 31.9,37.72 39.88,37.72 40.77,38.61 40.77,40.77 41.16,41.16 41.24,41.16 42.13,42.04 42.13,43.66 43.59,45.12 45.16,45.12 45.26,45.21 J11.3
D+
  Top 0.152: U6.29 9.99,27.01 9.65,26.67 9.65,19.16 10.3,19.16 10.54,18.92 10.54,18.16 10.42,18.04 8.54,18.04 D1.4
D-  (via drill 0.35)
  Top 0.152: U6.28 11.12,28.07 9.02,28.07 8.64,27.69 v8.64,25.53 | D1.6 7.2,18.39 7.2,18.63 7.11,18.72 7.11,19.05 7.11,19.49 v6.84,19.76
  Bottom 0.152: v8.64,25.53 8.64,21.97 8.1,21.43 7.5,21.43 6.64,20.58 6.64,19.96 v6.84,19.76
DCD  (via drill 0.35)
  Top 0.152: U6.8 26.41,35.63 26.94,35.1 26.94,33 v28.19,31.75 | v44.7,35.56 48.11,38.96 49.12,38.96 50.42,40.26 50.42,41.53 49.28,42.67 J10.2
  Bottom 0.152: v28.19,31.75 28.86,32.41 29.92,32.41 34.03,36.52 43.74,36.52 v44.7,35.56
DSR  (via drill 0.35)
  Top 0.152: J10.1 45.34,36.83 v44.7,36.83 | v29.08,33.02 28.61,33.49 U6.6
  Bottom 0.152: v44.7,36.83 33.91,36.83 30.1,33.02 v29.08,33.02
DTR  (via drill 0.35)
  Top 0.152: v25.4,33.02 25.4,33.8 25.39,33.81 25.39,36.09 U6.9 | v43.43,39.37 43.43,41.27 44.11,41.94 44.59,42.42 JP7.2
  Top 0.305: JP7.2 J11.2
  Bottom 0.152: v43.43,39.37 43.43,39.24 41.63,37.44 33.66,37.44 30.15,33.93 27.71,33.93 26.8,33.02 v25.4,33.02
GND  (via drill 0.35)  (3 unrouted)
  Top 0.152: U5.2 6.67,42.83 6.67,42.58 7.2,42.05 C6.2 7.15,40.89 R5.1 5.5,36.26 J7.1 | U4.2 23.87,40.78 23.87,39.98 25.65,38.2 25.65,38.1 v25.78,38.1 | JP7.1 44.03,43.16 44.03,43.4 44.47,43.84 49.12,43.84 49.78,43.18 v50,43.39 | U6.3 32.38,35.69 32.38,35.31 32.52,35.18 33.51,35.18 33.64,35.31 33.64,35.69 U6.1 34.36,35.92 v36.32,35.92 | U3.7 33.96,39.37 v34.54,39.37 | U2.EP 13.59,17.4 14.29,18.1 14.44,18.1 U2.4 14.44,18.64 C2.2 | C3.2 16.38,19.68 16.51,19.81 v16.45,19.88 | 30.17,6.13 C14.2 30.23,5.08 v29.97,4.83 | U6.32 11.41,23.96 U6.96 | D1.2 7.89,17.33 7.89,17.1 8.38,16.61 8.38,16.47 v8.43,16.43 | v7.68,14.8 6.44,16.04 6.44,16.61 5.94,17.11 J1.GND | U6.22 12.61,34.71 U6.91 | U6.30 11.31,26.06 U6.95 | U6.50 31.29,22.73 31.29,23.11 31.56,23.38 U6.76 | 15.07,11.44 U1.2 14.86,11.41 14.28,10.82 14.25,10.82 v13.84,10.41 | v15.23,9.14 16.8,9.14 R3.1
  Route2 0.152: v34.54,39.37 34.54,38.1 36.32,36.32 v36.32,35.92
  Bottom 0.152: v25.78,38.1 v25.78,41.4 | v50,43.39 52.11,43.39 52.32,43.18 v52.1,43.18 | v16.45,19.88 14.67,19.88 | v8.43,16.43 8.43,15.66 7.62,14.86 v7.68,14.8 | v13.84,10.41 14.48,10.41 15.49,9.4 v15.24,9.14 v15.23,9.14 | v29.97,4.83 32,2.79 B1.GND@0
  pour Top: 0.25,53.34 0.25,0 72.64,0 72.64,53.34
  pour Bottom: 0.25,53.34 0.25,0 72.64,0 72.64,53.34
GPIO1  (via drill 0.35)
  Top 0.152: v17.78,34.04 17.78,35.99 U6.16
  Top 0.406: R8.1 2.39,28.85 v2.79,28.85
  Route2 0.152: v2.79,28.85 15.34,28.85 15.95,29.46 15.95,38.44 15.65,38.74 15.65,39.24 16,39.6 16.51,39.6 16.86,39.24 16.86,39.02 17.78,38.1 v17.78,34.04
GPIO2
  Top 0.152: R5.2 7.2,39.52 7.98,40.3 7.98,42.47 U5.3
  Top 0.305: R5.2 7.2,34.96 8.55,33.61 U6.23
GPIO3_QWIIC  (via drill 0.35)
  Top 0.152: U3.13 30.32,43.78 v30.1,43.56
  Bottom 0.152: J6.1 7.9,31.27 9.27,31.27 10.64,32.64 10.67,32.64 10.67,34.04 9.65,35.05 9.65,36.2 10.92,37.47 22.71,37.47 22.86,37.31 23.62,37.31 24.15,37.85 24.15,38.12 24.26,38.23 24.26,43.31 24.51,43.56 v30.1,43.56
GPS_3.3V  (via drill 0.35)
  Top 0.152: C7.1 5.27,47.52 U5.5 4.22,45.88 4.06,45.72 v4.06,38.1 | J7.2 6.14,34.92 6.75,35.52 6.75,36.31 6.52,36.54 v6.52,36.96
  Bottom 0.152: v4.06,38.1 6.1,38.1 6.73,37.47 6.73,37.17 v6.52,36.96
HARDRX_ARDUINO
  Top 0.305: S1.3 45.01,45.5 45.97,46.46 50.52,46.46 B1.RX
HARDTX_ARDUINO  (via drill 0.35)
  Top 0.152: v44.7,38.1 43.36,38.1 S1.6
  Bottom 0.152: v44.7,38.1 49.53,38.1 52.7,41.27 52.7,50.42 B1.TX
IOREF  (via drill 0.35)
  Top 0.152: J4.4 v3.3,45.21 | v26.92,48.13 27.05,48.01 C4.1 | JP1.2 32,5.08 v32,6.35
  Top 0.305: C4.1 27.27,45.59 | 27.27,45.59 U3.14 | U4.7 23.82,44.27 23.82,44.7 24.72,45.59 27.27,45.59
  Bottom 0.152: v3.3,45.21 6.1,45.21 9.14,48.26 26.92,48.26 v26.92,48.13 27.66,48.87 32.25,48.87 32.35,48.77 38.23,48.77 40.39,46.61 40.39,44.19 41.24,44.19 42.13,43.3 42.13,41.24 38.63,37.74 33.53,37.74 30.02,34.24 25.76,34.24 24.79,33.27 24.79,33.17 24,32.38 24,14.35 v32,6.35 33.4,6.35 35.81,3.94 35.81,1.91 35.28,1.37 29.95,1.37 29.46,1.37 23.9,1.37 22.73,2.54 B1.IOREF
N$1
  Top 0.152: J1.D- 5.43,18.84 6.18,18.84 6.51,18.51 6.89,18.51 6.89,17.96 7.25,17.61 D1.1
N$3
  Top 0.152: J1.D+ 5.43,18.19 6.18,18.19 6.31,18.06 6.31,17.68 8.25,15.75 9.53,15.75 10.03,16.26 10.03,17.27 9.78,17.53 8.3,17.53 D1.3
N$4
  Top 0.152: D4.A 5.63,23.37 R4.1
N$6  (via drill 0.35)
  Top 0.152: v8.61,20.2 8.89,20.49 8.89,24.26 8.38,24.77 R1.2 | v10.41,12.7 11.46,11.65 U1.1
  Bottom 0.152: v8.61,20.2 9.72,19.09 9.72,18.66 10.72,17.67 10.72,16.05 11.02,15.74 11.02,14.58 10.41,13.97 v10.41,12.7
N$7
  Top 0.152: D2.C R1.1
N$8
  Top 0.305: U6.62 40.22,32.51 R6.1
N$9
  Top 0.152: B1.D5 JP2.1
N$10
  Top 0.152: R2.2 13.84,14.19 U1.5
N$11
  Top 0.152: B1.D6 JP3.1
N$12
  Top 0.305: U6.56 C18.1
N$13
  Top 0.305: C19.1 43.69,25.95 L1.1 41.62,25.91 C18.2
N$14
  Top 0.305: L2.2 47.37,27.85 C20.1 R6.2
N$15
  Top 0.305: JP4.1 51.18,19.81 49.12,21.87 JP5.1 47.41,25.91 L2.1 47.33,25.91 C19.2
N$16
  Top 0.152: 59.02,19.81 JP4.2
  Top 1.27: E1.FEED 59.07,19.76 59.02,19.81
N$17
  Top 0.152: D6.C 5.63,26.16 R7.2
N$18
  Top 0.152: JP5.2 J9.FEED
N$19
  Top 0.152: R8.2 3.16,29.81 Q2.1
N$20
  Top 0.152: Q2.3 7.45,26.67 R7.1
PWR_ON
  Top 0.152: S3.3 18.71,43.9 U6.15
RESET_N
  Top 0.152: S4.3 12.06,46.74 15.37,46.74 15.62,46.48 15.62,36.37 U6.18
RI  (via drill 0.35)
  Top 0.152: J11.1 45.59,39.24 44.7,39.24 v44.7,39.37 | v28.17,33.02 27.51,33.68 U6.7
  Bottom 0.152: v44.7,39.37 42.47,37.13 33.78,37.13 30.28,33.63 28.83,33.63 28.23,33.02 v28.17,33.02
RTS
  Top 0.152: J10.3 JP6.2 50.41,44.84 50.8,44.45 50.8,40.01 49.15,38.35 48.26,38.35 45.59,35.69 45.59,34.92 45.21,34.54 44.2,34.54 43.81,34.92 43.81,35.94 42.42,37.34 31.85,37.34 31.11,38.07 30.61,38.07 29.68,37.14 24.82,37.14 24.69,37.01 24.69,36.63 U6.10
RX_ARDUINO  (via drill 0.35)
  Top 0.152: J4.2 30.23,49.15 30.99,48.39 30.99,45.6 U3.12 30.97,44.08 v31.5,43.56 | v39.12,43.81 S1.2
  Bottom 0.152: v31.5,43.56 36.36,43.56 36.99,44.19 38.24,44.19 38.62,43.81 v39.12,43.81
RX_CELL  (via drill 0.35)
  Top 0.152: U3.4 31.35,39.48 31.35,39.16 30.87,38.68 30.36,38.68 29.9,38.23 v28.58,38.23 | v21.84,32.89 20.91,33.82 U6.13
  Bottom 0.152: v28.58,38.23 23.24,32.89 v21.84,32.89
SCL_CELL  (via drill 0.35)
  Top 0.152: U4.5 26.02,42.93 26.04,42.93 v26.04,42.95 | v8.76,29.45 10.92,29.45 U6.27
  Bottom 0.152: v26.04,42.95 26.04,42.01 26.39,41.65 26.39,37.85 25.25,36.71 22.99,36.71 15.49,29.21 9.4,29.21 9.15,29.45 v8.76,29.45
SCL_QWIIC  (via drill 0.35)
  Top 0.152: J5.2 4.04,32.92 J7.4 7.6,32.92 8.64,31.88 v9.02,31.88 | v23.75,46.1 23.25,45.6 U4.8
  Bottom 0.152: v9.02,31.88 9.4,31.88 10.11,32.59 10.11,33.33 9.32,34.11 9.32,36.32 10.84,37.85 22.76,37.85 22.99,37.62 23.49,37.62 23.85,37.98 23.85,38.48 23.81,38.51 23.81,40.64 23.81,46.04 v23.75,46.1
SDA_CELL  (via drill 0.35)
  Top 0.152: U4.4 24.75,42.15 v25.02,42.42 | v9.14,30.35 11.12,30.35 U6.26
  Bottom 0.152: v25.02,42.42 25.02,38.28 23.75,37.01 22.41,37.01 15.75,30.35 v9.14,30.35
SDA_QWIIC  (via drill 0.35)
  Top 0.152: J5.1 4.06,35.43 4.06,34.31 4.29,34.31 4.69,33.92 J7.3 7.48,33.92 8.51,32.89 v9.02,32.89 | v23.24,38.23 23.24,40.88 U4.1
  Bottom 0.152: v9.02,32.89 9.02,36.45 10.79,38.23 v23.24,38.23
SHIELD  (2 unrouted)
  Top 0.152: J1.SHIELD8 2.53,21.09 J1.SHIELD3 J1.SHIELD4 2.63,17.35 J1.SHIELD6 2.79,15.71 | J1.SHIELD 5.31,21.15 | J1.SHIELD2 5.28,15.71 2.79,15.71 | J1.SHIELD8 2.48,16.03 2.79,15.71 | J1.SHIELD8 2.79,21.15
  Top 0.406: 2.79,21.15 5.31,21.15
  Bottom 0.152: J1.SHIELD9 2.98,20.84 J1.SHIELD5 | J1.SHIELD10 5.1,15.69 J1.SHIELD7
SIM_CLK  (via drill 0.35)
  Top 0.152: J8.C3 22.23,12.06 v22.35,12.19 24,12.19 24.64,11.56 C16.1 | v20.83,20 17.72,20 17.53,20.19 17.53,22.17 U6.38 | D5.6 34.7,6.71 34.98,6.71 35.58,7.31 v35.58,9.4
  Route2 0.152: v20.83,20 20.83,20.07 21.72,20.07 21.97,19.81 21.97,13.94 21.75,13.71 21.75,13.21 22.35,12.6 v22.35,12.19 22.99,11.56 22.99,10.85 24.38,9.45 33.96,9.45 34.06,9.55 34.06,9.65 34.42,10.01 34.92,10.01 35.28,9.65 35.28,9.55 35.43,9.4 v35.58,9.4
SIM_IO  (via drill 0.35)
  Top 0.152: U6.39 18.71,20.66 18.8,20.57 v18.8,20.6 | J8.C7 22.1,10.79 v22.35,11.05 22.73,11.05 23.11,10.67 C15.1 | v34.67,9.4 34.67,8.58 D5.4
  Route2 0.152: v18.8,20.6 20.19,19.2 20.19,11.56 20.32,11.43 22.23,11.43 22.35,11.3 v22.35,11.05 24.26,9.14 34.67,9.14 v34.67,9.4
SIM_RST  (via drill 0.35)
  Top 0.152: J8.C2 22.23,13.34 v22.35,13.46 23.83,13.46 26.04,11.25 26.04,8.82 26.16,8.7 C17.1 | v22.42,20.6 20.29,20.6 19.81,21.08 U6.40 | v36.49,9.4 36.58,9.3 D5.3
  Route2 0.152: v22.42,20.6 22.42,20.64 22.86,21.08 23.24,21.08 23.37,20.95 23.37,18.29 22.35,17.27 v22.35,13.46 22.35,13.05 23.29,12.11 23.29,11 24.51,9.78 33.76,9.78 34.29,10.31 35.52,10.31 36.44,9.4 v36.49,9.4
SOFTRX_ARDUINO
  Top 0.305: B1.D8 36.62,47.46 S1.1
SOFTTX_ARDUINO
  Top 0.305: B1.D9 34.8,46.74 34.8,40.64 35.59,39.85 S1.4
TX_ARDUINO  (via drill 0.35)
  Top 0.152: J4.3 4.32,48.77 27.94,48.77 28.19,48.51 v28.19,48.26 | v32,48.26 32,46.99 31.75,46.74 31.62,46.74 U3.11 | v37.85,46.99 37.85,45.05 36.1,43.3 36.1,42.04 36.99,41.16 37.81,41.16 S1.5
  Bottom 0.152: v28.19,48.26 v32,48.26 37.46,48.26 37.85,47.88 v37.85,46.99
TX_CELL  (via drill 0.35)
  Top 0.152: U3.3 30.7,39.48 30.7,39.16 30.57,39.03 28.52,39.03 27.72,38.23 v27.3,38.23 | v21.97,34.16 21.97,36.12 U6.12
  Bottom 0.152: v27.3,38.23 23.24,34.16 v21.97,34.16
V_BATT
  Top 0.152: Q1.3 16.81,12.7 16.36,12.24 16.36,12.2 U1.3 15.81,11.15 C1.1 11.66,11.03 J2.2
  Top 0.406: J3.2 7.75,11.3 J2.2
V_USB  (via drill 0.35)
  Top 0.152: 19.03,8.62 R3.2 19.31,8.94 D3.A 19.94,10.91 19.94,13.34 19.69,13.59 17.1,13.59 Q1.1 16.43,14.25 U1.4 14.57,15.49 v10.41,15.49 | 19.03,8.62 21.34,6.31 JP8.1 | S2.1 12.83,7.27 v12.83,7.24 | v18.54,6.99 19.03,7.47 19.03,8.62 | J1.VBUS 5.58,20.09 6.31,20.09 6.53,20.31 6.53,21.59 | 6.53,21.59 6.53,26.88 6.4,27.02 3.04,27.02 2.69,26.67 2.69,25.79 D2.A | D1.5 v7.75,19.68 7.75,19.97 7.14,20.58 7.14,20.98 6.53,21.59
  Top 0.406: S2.4 10.06,1.62 10.03,1.65 10.03,7.24 10.06,7.27 S2.1
  Bottom 0.152: v12.83,7.24 15.88,7.24 16.13,6.99 v18.54,6.99 | v10.41,15.49 10.41,17.54 9.42,18.54 9.42,18.78 9.14,19.05 8.38,19.05 v7.75,19.68
VIN  (via drill 0.35)
  Top 0.152: U2.8 11.69,16.7 11.54,16.7 11.41,16.83 11.41,17.97 11.54,18.1 11.69,18.1 U2.5 12.48,18.9 | C2.1 12.74,18.9 12.48,18.9 | v18.16,11.68 18.1,11.75 Q1.2 17.01,11.73 D3.C 17.53,10.29 18.16,9.65 18.16,8.11 17.96,7.91 17.23,7.91 S2.3 | v11.56,19.18 11.84,18.9 12.48,18.9
  Top 0.406: S2.6 16.6,3.12 17.24,3.76 17.24,5.13 16.6,5.77 S2.3
  Bottom 0.152: v18.16,11.68 13.33,16.51 12.12,16.51 11.18,17.45 11.18,18.92 11.43,19.18 v11.56,19.18
VSIM  (via drill 0.35)
  Top 0.152: C14.1 C13.1 27.47,8.81 26.48,8.81 26.35,8.95 26.35,11.37 23.37,14.35 v23.37,15.49 | U6.41 21.39,21.79 21.39,21.41 21.59,21.21 23.37,21.21 23.62,20.95 23.62,17.4 v23.4,17.4 | v23.37,15.49 22.99,15.49 22.61,15.88 J8.C1 | v23.37,15.49 31.91,6.96 32.39,6.96 33.59,5.76 34.98,5.76 35.51,6.29 D5.1
  Bottom 0.152: v23.4,17.4 23.4,15.52 v23.37,15.49
VUSB_DET  (via drill 0.35)
  Top 0.152: JP8.2 19.73,4.67 v19.32,5.09 | U6.17 16.51,38.73 v16.26,38.99
  Route2 0.152: v16.26,38.99 16.26,20.54 15.84,20.13 15.84,8.57 v19.32,5.09

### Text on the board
tNames: LTE 4G Nano-Sim / IoT Module | gautamk97

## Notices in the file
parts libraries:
SparkFun-Connectors: Licensing: Creative Commons ShareAlike 4.0 International - https://creativecommons.org/licenses/by-sa/4.0
